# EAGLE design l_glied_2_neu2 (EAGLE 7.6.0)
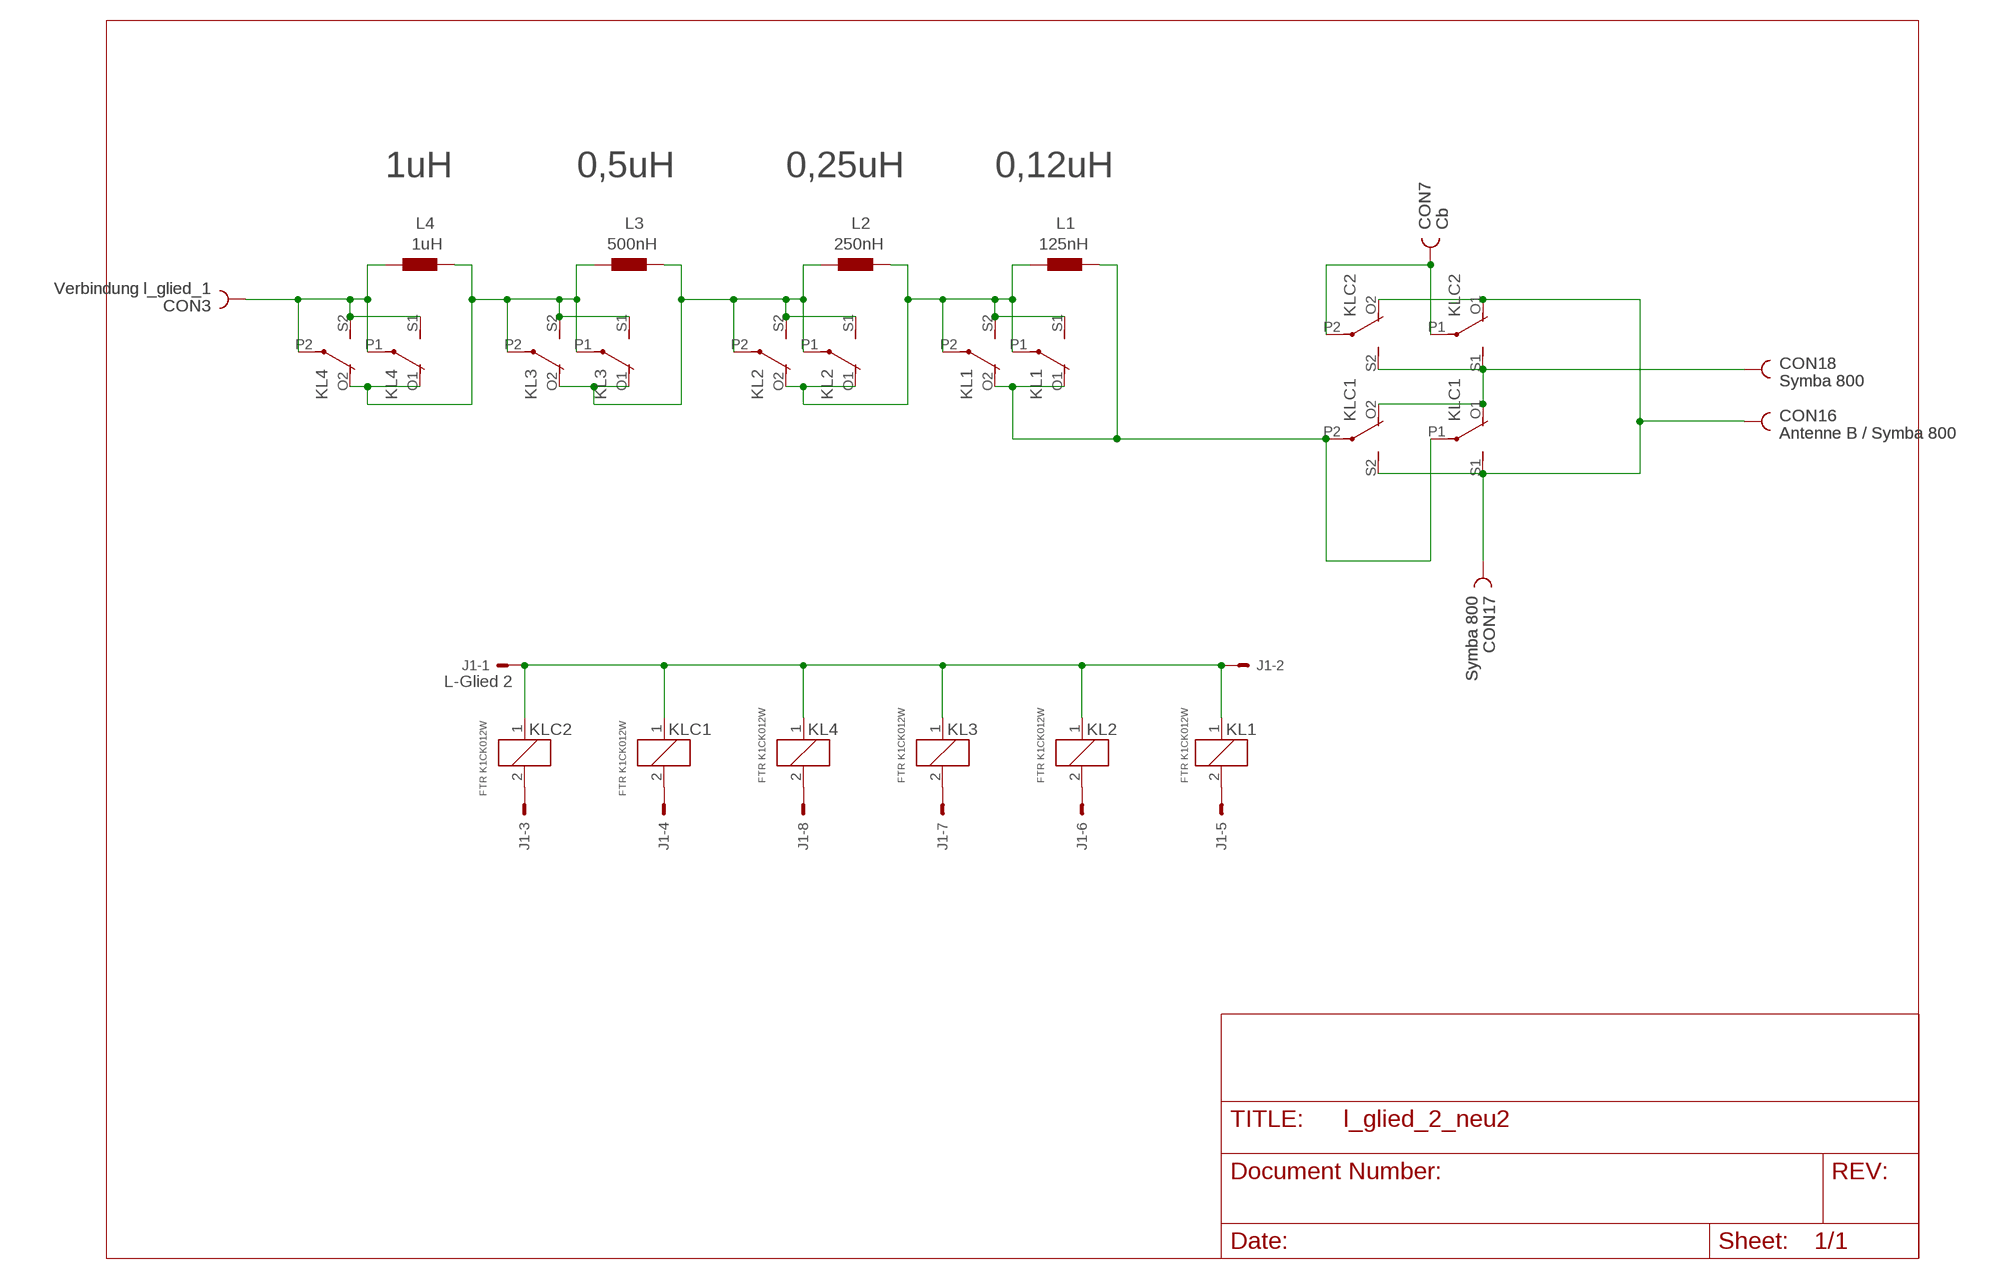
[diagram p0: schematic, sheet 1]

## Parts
CON3  Verbindung l_glied_1  PIN2_53MM  [HOLE3]
CON7  Cb  PIN2_53MM  [HOLE3]
CON16  Antenne B / Symba 800  PIN2_53MM  [HOLE3]
CON17  Symba 800  PIN2_53MM  [HOLE3]
CON18  Symba 800  PIN2_53MM  [HOLE3]
J1  L-Glied 2  22-27-2081-08  [6410-08]
KL1  FTR K1CK012W  4052  [F4052]
KL2  FTR K1CK012W  4052  [F4052]
KL3  FTR K1CK012W  4052  [F4052]
KL4  FTR K1CK012W  4052  [F4052]
KLC1  FTR K1CK012W  4052  [F4052]
KLC2  FTR K1CK012W  4052  [F4052]
L1  125nH  INDUKT13X10  [L_13X10]
L2  250nH  INDUKT17X10  [L_17X10]
L3  500nH  INDUKT15X15  [L_15X15]
L4  1uH  INDUKT24X15  [L_24X15]

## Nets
N$1: KL1.O1(2:O) KL1.O2(3:O) KLC1.P1(2:P) KLC1.P2(3:P) L1.P$2
N$2: J1.6 KL2.2
N$3: J1.7 KL3.2
N$4: J1.5 KL1.2
N$5: J1.1 J1.2 KL1.1 KL2.1 KL3.1 KL4.1 KLC1.1 KLC2.1
N$7: J1.3 KLC2.2
N$8: J1.8 KL4.2
N$10: CON16.1 CON17.1 KLC1.S1(2:S) KLC1.S2(3:S) KLC2.O1(2:O) KLC2.O2(3:O)
N$11: CON18.1 KLC1.O1(2:O) KLC1.O2(3:O) KLC2.S1(2:S) KLC2.S2(3:S)
N$12: J1.4 KLC1.2
N$15: CON7.1 KLC2.P1(2:P) KLC2.P2(3:P)
N$24: KL1.P1(2:P) KL1.P2(3:P) KL1.S1(2:S) KL1.S2(3:S) KL2.O1(2:O) KL2.O2(3:O) L1.P$1 L2.P$2
N$27: KL3.P1(2:P) KL3.P2(3:P) KL3.S1(2:S) KL3.S2(3:S) KL4.O1(2:O) KL4.O2(3:O) L3.P$1 L4.P$2
N$33: CON3.1 KL4.P1(2:P) KL4.P2(3:P) KL4.S1(2:S) KL4.S2(3:S) L4.P$1
N$40: KL2.P1(2:P) KL2.P2(3:P) KL2.S1(2:S) KL2.S2(3:S) KL3.O1(2:O) KL3.O2(3:O) L2.P$1 L3.P$2

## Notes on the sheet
- 1uH | 0,5uH | 0,25uH | 0,12uH

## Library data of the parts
CON3 CON7 CON16-CON18 = lindenau:PIN2_5
J1 = con-molex:22-?-08: CONNECTOR wire to board 2.54 mm (.1 inch) pitch header; OC_FARNELL: unknown; OC_NEWARK: unknown
KL1-KL4 KLC1 KLC2 = relay:4052: RELAY 2 x switch, Finder; OC_FARNELL: unknown; OC_NEWARK: unknown
L1-L4 = lindenau:INDUKT

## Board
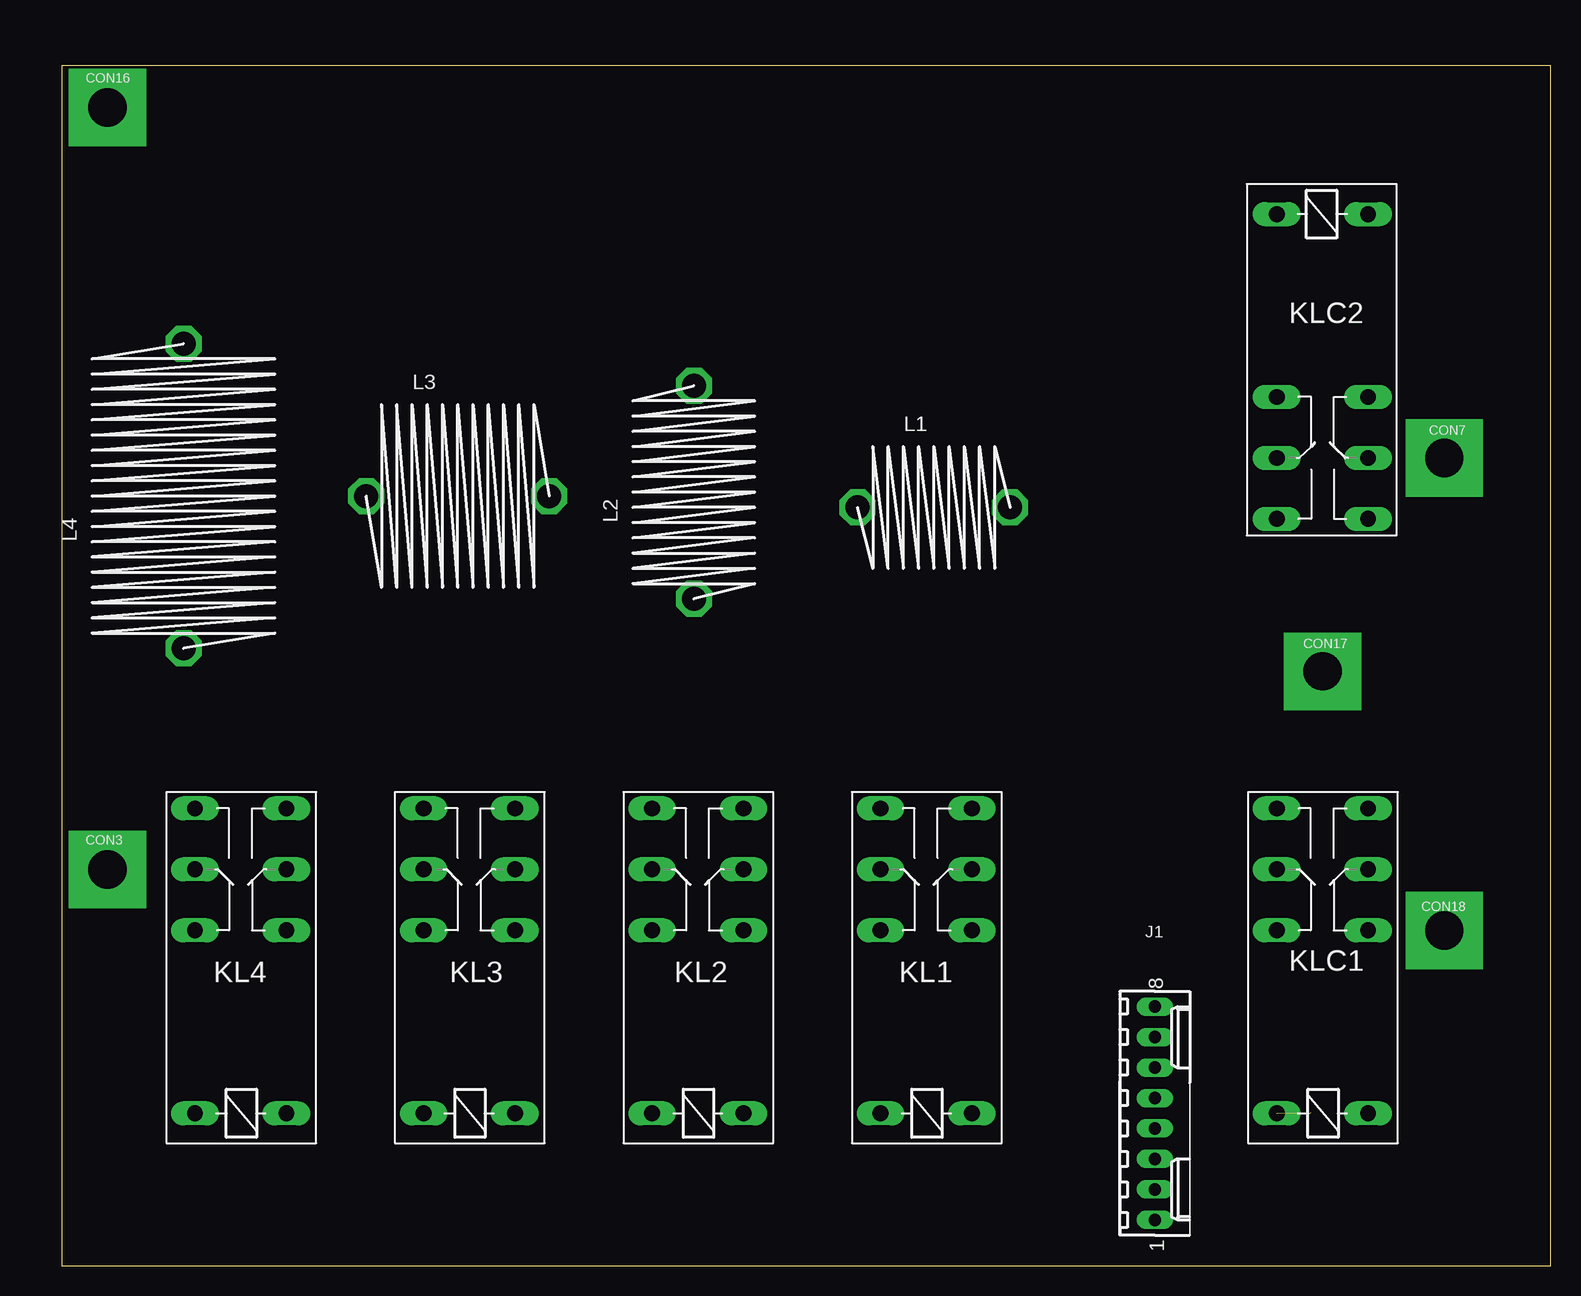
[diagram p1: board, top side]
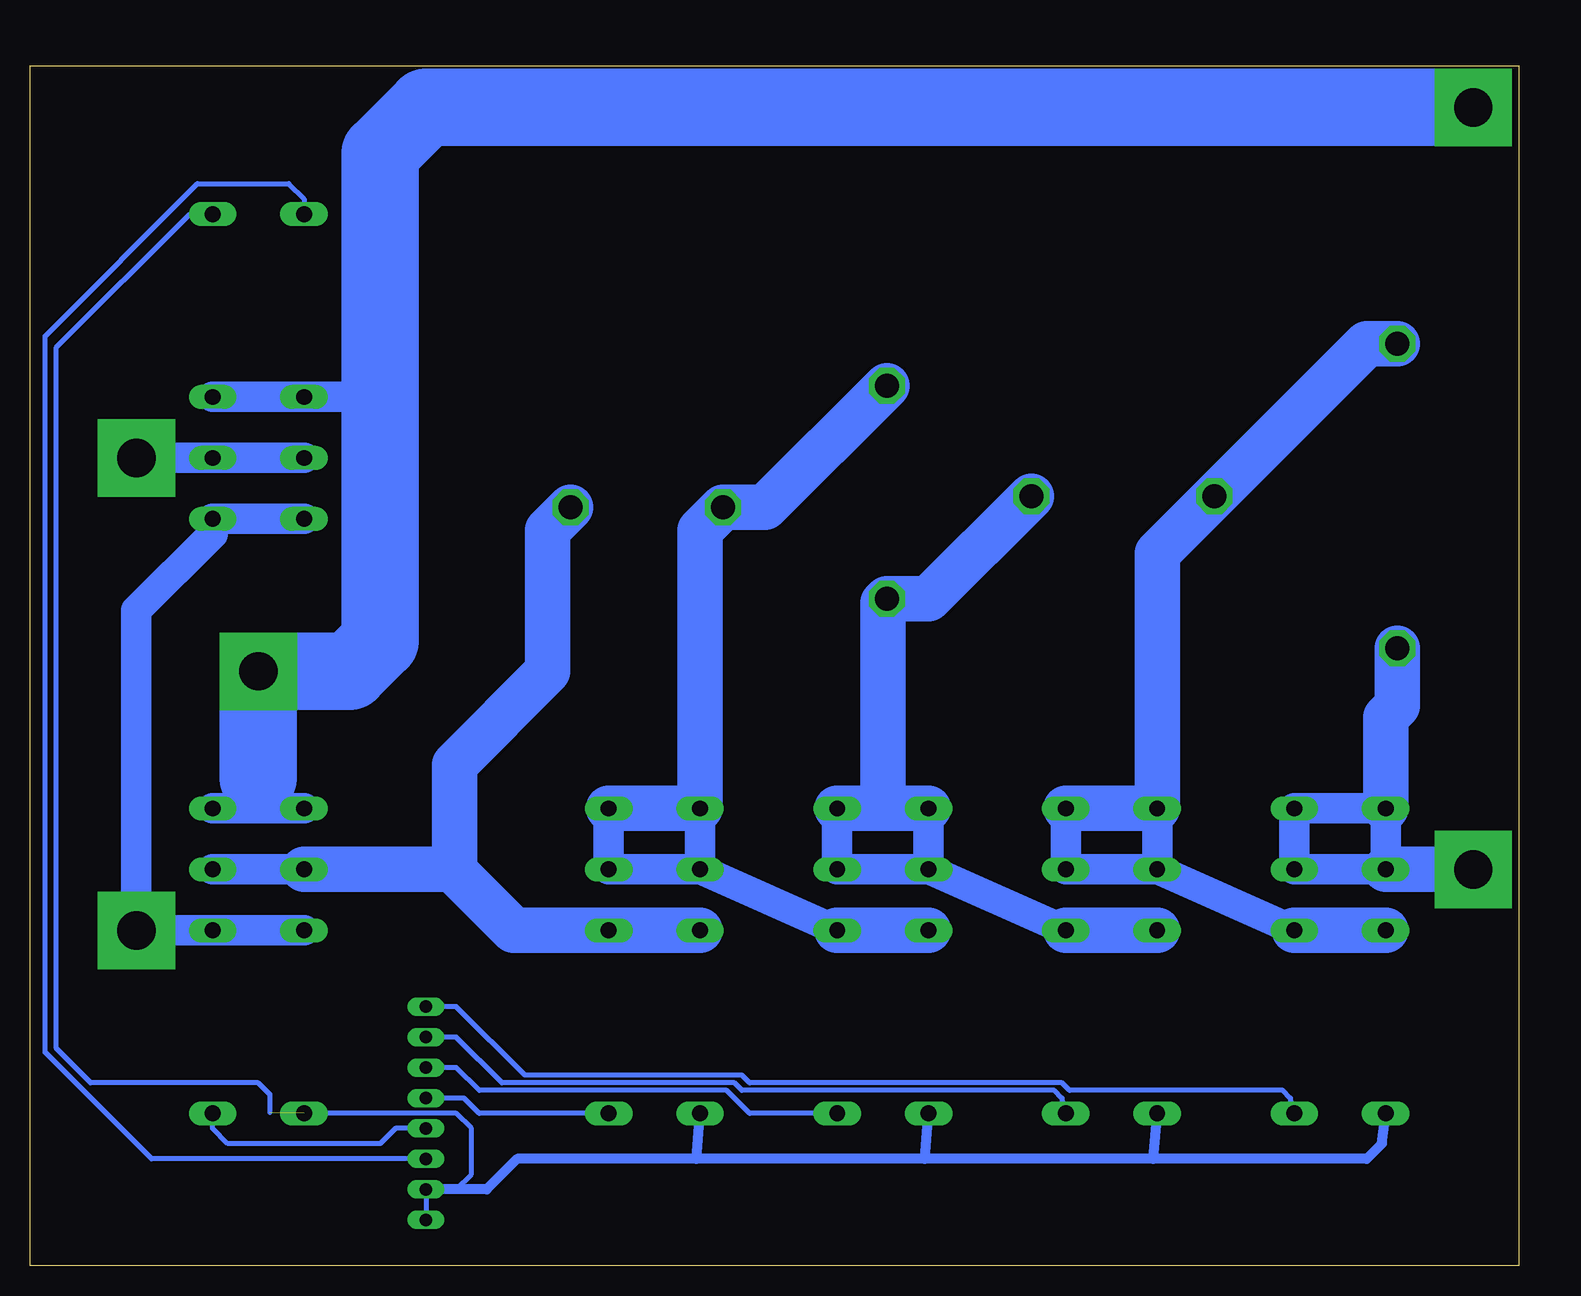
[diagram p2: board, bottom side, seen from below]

Size 124.12 x 100 mm. Coordinates in mm from the lower left corner, seen from the top.
Outline: 0,0 124.12,0 124.12,100 0,100 0,0
Copper layers (1*16): Top 0.035mm / dielectric 1.5mm / Bottom 0.035mm
Design rules "default": minimum track width 10mil, minimum drill 24mil, track to track 8mil, track to pad 8mil, pad to pad 8mil, via to via 8mil, smd to smd 8mil, copper to edge 40mil, drill to drill 8mil, minimum pad ring 10mil, minimum via ring 8mil, stop-mask expansion 4mil, vias tented up to drill 0mil, thermal gap 10mil

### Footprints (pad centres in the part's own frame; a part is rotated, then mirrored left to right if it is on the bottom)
HOLE3 = drill 3.2 pad 6.452 square: 1 0,0
6410-08 = drill 1.016 long: 1 8.89,0; 2 6.35,0; 3 3.81,0; 4 1.27,0; 5 -1.27,0; 6 -3.81,0; 7 -6.35,0; 8 -8.89,0
F4052 = drill 1.321 long: 1 -3.81,3.81; 2 -3.81,-3.81; O1 11.43,-3.81; O2 11.43,3.81; P1 16.51,-3.81; P2 16.51,3.81; S1 21.59,-3.81; S2 21.59,3.81
L_13X10 = drill 2 octagon: P$1 -6.35,0; P$2 6.35,0
L_17X10 = drill 2 octagon: P$1 -8.89,0; P$2 8.89,0
L_15X15 = drill 2 octagon: P$1 -7.62,0; P$2 7.62,0
L_24X15 = drill 2 octagon: P$1 -12.7,0; P$2 12.7,0

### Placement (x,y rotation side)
CON3  3.81,33.02 0 top
CON7  115.25,67.31 0 top
CON16  3.81,96.52 0 top
CON17  105.09,49.53 0 top
CON18  115.25,27.94 0 top
J1  91.12,12.7 270 top
KL1  72.07,16.51 90 top
KL2  53.02,16.51 90 top
KL3  33.97,16.51 90 top
KL4  14.92,16.51 90 top
KLC1  105.09,16.51 90 top
KLC2  105.09,83.82 270 top
L1  72.71,63.18 0 top
L2  52.7,64.45 90 top
L3  33.02,64.14 0 top
L4  10.16,64.14 90 top

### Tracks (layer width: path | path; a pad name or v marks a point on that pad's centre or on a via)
N$1
  Bottom 2.54: KLC1.P2 KLC1.P1
  Bottom 3.81: KL1.O2 KL1.O1 83.82,27.94 88.74,32.86 | 88.74,32.86 88.9,33.02 KLC1.P2 | L1.P$2 80.96,61.28 80.96,49.53 88.74,41.75 88.74,32.86
N$2
  Bottom 0.406: KL2.2 64.14,12.7 66.04,14.61 86.68,14.61 88.58,16.51 J1.6
N$3
  Bottom 0.406: KL3.2 38.1,13.97 38.73,14.61 64.77,14.61 65.41,15.24 84.77,15.24 88.58,19.05 J1.7
N$4
  Bottom 0.406: KL1.2 86.68,12.7 87.95,13.97 J1.5
N$5  (1 unrouted)
  Bottom 0.406: KLC1.1 88.58,12.7 87.31,11.43 87.31,7.62 88.58,6.35 J1.2 J1.1 | KLC2.1 110.81,87.63 121.92,76.52 121.92,18.1 119.06,15.24 105.09,15.24 104.14,14.29 104.14,12.75
  Bottom 0.813: J1.2 86.04,6.35 83.5,8.89 68.58,8.89 | 30.48,8.89 12.7,8.89 11.43,10.16 KL4.1 | 30.48,8.89 49.53,8.89 | 49.53,8.89 68.58,8.89 | 30.48,8.89 KL3.1 | 49.53,8.89 KL2.1 | 68.58,8.89 KL1.1
N$7
  Bottom 0.406: KLC2.2 101.28,88.9 102.55,90.17 110.17,90.17 122.87,77.47 122.87,17.78 113.98,8.89 J1.3
N$8
  Bottom 0.406: KL4.2 19.05,13.97 19.68,14.61 37.47,14.61 38.1,15.24 64.14,15.24 64.77,15.88 82.87,15.88 88.58,21.59 J1.8
N$10
  Bottom 2.54: 105.09,38.1 KLC1.S2 | 105.09,38.1 KLC1.S1 | 105.09,40.64 105.09,38.1 | KLC2.O2 KLC2.O1 94.93,72.39
  Bottom 6.452: 105.09,40.64 CON17.1 97.47,49.53 94.93,52.07 94.93,72.39 94.93,92.71 91.12,96.52 CON16.1
N$11
  Bottom 2.54: KLC1.O2 KLC1.O1 CON18.1 115.25,54.61 108.9,60.96 KLC2.S2 KLC2.S1
N$12
  Bottom 0.406: J1.4 93.66,11.43 94.93,10.16 107.63,10.16 108.9,11.43 KLC1.2
N$15
  Bottom 2.54: KLC2.P1 KLC2.P2 CON7.1
N$24
  Bottom 2.54: KL1.P2 KL1.P1 KL1.S1 | KL1.P2 KL1.S2 | KL2.O1 KL1.P2
  Bottom 3.81: KL2.O2 KL2.O1 | L2.P$2 62.87,63.18 L1.P$1 68.26,61.28 KL1.S2 KL1.S1
N$27
  Bottom 2.54: KL3.P2 KL3.S2 | KL3.P2 KL3.P1 KL3.S1 | KL4.O1 KL3.P2
  Bottom 3.81: KL4.O2 KL4.O1 | L4.P$2 12.7,76.83 L3.P$1 30.16,59.37 KL3.S2 KL3.S1
N$33
  Bottom 2.54: KL4.P2 KL4.P1 KL4.S1 KL4.S2 KL4.P2
  Bottom 3.81: CON3.1 KL4.P2 | L4.P$1 10.16,46.67 11.11,45.72 KL4.S2
N$40
  Bottom 2.54: KL2.P2 KL2.P1 KL2.S1 | KL2.P2 KL2.S2 | KL3.O1 KL2.P2
  Bottom 3.81: KL3.O2 KL3.O1 | 53.02,38.1 KL2.S2 | L3.P$2 49.21,55.56 L2.P$1 53.02,55.24 53.02,38.1 | 53.02,38.1 KL2.S1

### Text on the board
Document: Rel. KL4 | Rel. KL3 | Rel. KL2 | Rel. KL1 | Rel. KLC1 | Rel. KLC2 | 12 Volt | 12 Volt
